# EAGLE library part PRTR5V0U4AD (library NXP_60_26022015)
ESD protection AAL Eindhoven MK
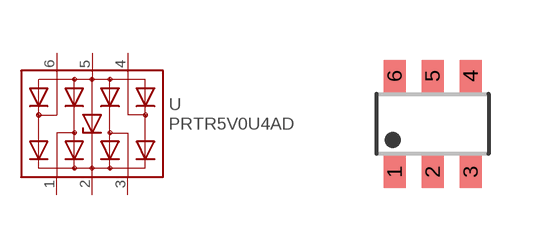
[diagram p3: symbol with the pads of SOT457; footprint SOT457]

Designator prefix U

## PRTR5V0U4AD (FARNELL: 1757868)  [SOT457]
1  ESD1  pas
2  VCC  pwr
3  ESD2  pas
4  ESD3  pas
5  GND  pwr
6  ESD4  pas

## Footprint SOT457 (pad centres in mm)
SOT457 TSOP6: Plastic surface-mounted package; 6 lead JEIDA: SC73 A.K.A. SOT23-6
smd 0.55 x 0.8: 1 -0.95,-1.2; 2 0,-1.2; 3 0.95,-1.2; 4 0.95,1.2; 5 0,1.2; 6 -0.95,1.2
